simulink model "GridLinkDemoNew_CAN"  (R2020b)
settings: Solver=FixedStepDiscrete  StartTime=0.0  StopTime=inf  RelTol=1e-3  EnableMultiTasking=on
InitFcn:
  | clc
  | close all
  | f_mod = 50000;
  | f_mod1 = 50*1e3; %[12 24 36 48 72 84 96 144]*1e3; %[18 36 48 72 84 96 144]*1e3;%
  | 
  | 
  | %%
  | 
  | 
  |             Tmod1 = 1/f_mod1;
  |             Tmod = 1/f_mod;
  |             Tc = Tmod1;
  |             Tsw=Tc;
  | 
  | warning off
  | f_sig = 60;
  | 
  | U_ac = 10;
  | U_dc = 20;
  | Ts= 0.01*Tsw;
  | 
  | Fc=50000
  | Fc1=1000
  | 
  | 
  | CounterCut_Outer=2000
  | 
  | 
  | INNER_PWM=1000
  | OUTER_PWM=50000
undefined symbols (not defined in the file): A, ADCIN0, ADCIN1, ADCINA0, ADCINB0, bit, Compare, conversion, DCAEVT1, DCAEVT1FILT, Digital, Down, ended, Event, Filtered, GPTRIP1SEL, GPTRIP2SEL, hex2dec, identifier, input, Module, Newinv, of, Single, SPS_EMT_TAPAS_2018b, Standard, start, Trip, TZ1, TZ2, Up, version, Zone
libraries: tiiqmathlib x63, c2802xlib x25, c2837xDlib x5, c280xlib x5, c28xdmclib x2, svdutilitieslib x1, c2000lib x1, canmsglib x1, simulink x1
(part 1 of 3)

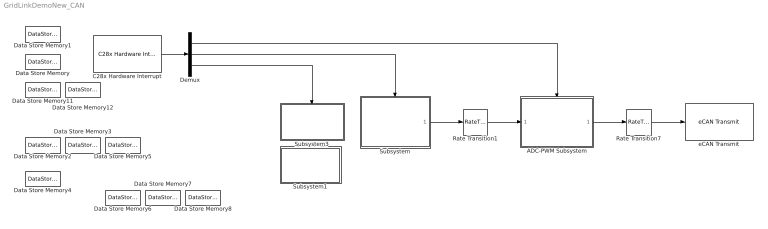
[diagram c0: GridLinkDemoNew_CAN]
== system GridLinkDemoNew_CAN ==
  ADC-PWM Subsystem : Subsystem  TreatAsAtomicUnit=on
  C28x Hardware Interrupt : c2000lib/Scheduling/C28x Hardware Interrupt  irqnumbers=[1 9 3]  pienumbers=[1 7 8]  irqpriorities=[30 10 20]  irqpreempts=[1 1 0]  showinput=off  dspchiptype=C280X
  Data Store Memory : DataStoreMemory  DataStoreName=Counter  ReadBeforeWriteMsg=warning  WriteAfterWriteMsg=warning  WriteAfterReadMsg=warning  ShowAdditionalParam=off
  Data Store Memory1 : DataStoreMemory  DataStoreName=CounterCut  ReadBeforeWriteMsg=warning  WriteAfterWriteMsg=warning  WriteAfterReadMsg=warning  InitialValue=2222  ShowAdditionalParam=off
  Data Store Memory11 : DataStoreMemory  DataStoreName=VdcP  ReadBeforeWriteMsg=warning  WriteAfterWriteMsg=warning  WriteAfterReadMsg=warning  InitialValue=2222  ShowAdditionalParam=off
  Data Store Memory12 : DataStoreMemory  DataStoreName=VdcN  ReadBeforeWriteMsg=warning  WriteAfterWriteMsg=warning  WriteAfterReadMsg=warning  InitialValue=2222  ShowAdditionalParam=off
  Data Store Memory2 : DataStoreMemory  DataStoreName=I_o_A  ReadBeforeWriteMsg=warning  WriteAfterWriteMsg=warning  WriteAfterReadMsg=warning  ShowAdditionalParam=off
  Data Store Memory3 : DataStoreMemory  DataStoreName=I_o_B  ReadBeforeWriteMsg=warning  WriteAfterWriteMsg=warning  WriteAfterReadMsg=warning  ShowAdditionalParam=off
  Data Store Memory4 : DataStoreMemory  DataStoreName=Temp_P1  ReadBeforeWriteMsg=warning  WriteAfterWriteMsg=warning  WriteAfterReadMsg=warning  ShowAdditionalParam=off
  Data Store Memory5 : DataStoreMemory  DataStoreName=I_o_C  ReadBeforeWriteMsg=warning  WriteAfterWriteMsg=warning  WriteAfterReadMsg=warning  ShowAdditionalParam=off
  Data Store Memory6 : DataStoreMemory  DataStoreName=I_s_A  ReadBeforeWriteMsg=warning  WriteAfterWriteMsg=warning  WriteAfterReadMsg=warning  ShowAdditionalParam=off
  Data Store Memory7 : DataStoreMemory  DataStoreName=I_s_B  ReadBeforeWriteMsg=warning  WriteAfterWriteMsg=warning  WriteAfterReadMsg=warning  ShowAdditionalParam=off
  Data Store Memory8 : DataStoreMemory  DataStoreName=I_s_C  ReadBeforeWriteMsg=warning  WriteAfterWriteMsg=warning  WriteAfterReadMsg=warning  ShowAdditionalParam=off
  Demux : Demux  Outputs=3
  Rate Transition1 : RateTransition  Deterministic=off
  Rate Transition7 : RateTransition  Deterministic=off  OutPortSampleTime=0.01
  Subsystem : Subsystem
  Subsystem1 : Subsystem
  Subsystem3 : Subsystem
  eCAN Transmit : c280xlib/eCAN Transmit  chipFamily=C280x  useModule=eCAN_B  mailboxNo=1  messageID=hex2dec('0x01B')  messageType=Standard (11-bit identifier)  enableBlockingMode=on  postInterrupt=off  interruptLine=0
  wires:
  Rate Transition1/1 -> ADC-PWM Subsystem/1(In1)
  ADC-PWM Subsystem/1(Out1) -> Rate Transition7/1
  Subsystem/1(Out3) -> Rate Transition1/1
  C28x Hardware Interrupt/1 -> Demux/1
  Rate Transition7/1 -> eCAN Transmit/1
  Demux/2 -> Subsystem/Trigger
  Demux/1 -> ADC-PWM Subsystem/Trigger
  Demux/3 -> Subsystem3/Trigger
